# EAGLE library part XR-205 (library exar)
Monolithic WAVEFORM GENERATOR
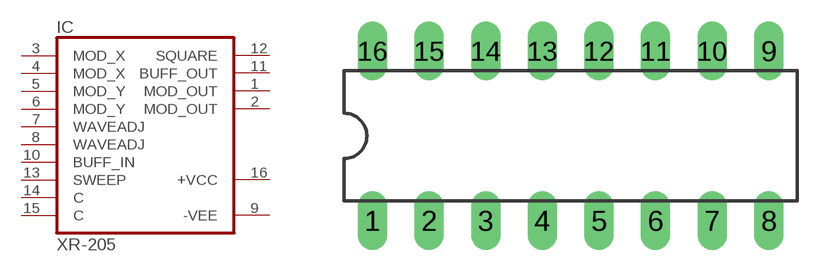
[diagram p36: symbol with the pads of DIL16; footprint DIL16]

Designator prefix IC

## XR-205 (OC_FARNELL: unknown; OC_NEWARK: unknown)  [DIL16]
1  MOD_OUT  out
2  MOD_OUT  out
3  MOD_X  in
4  MOD_X  in
5  MOD_Y  in
6  MOD_Y  in
7  WAVEADJ  in
8  WAVEADJ  in
9  -VEE  pwr
10  BUFF_IN  in
11  BUFF_OUT  out
12  SQUARE  out
13  SWEEP  in
14  C  in
15  C  in
16  +VCC  pwr

## Footprint DIL16 (pad centres in mm)
Dual In Line Package
drill 0.813 long: 1 -8.89,-3.81; 2 -6.35,-3.81; 3 -3.81,-3.81; 4 -1.27,-3.81; 5 1.27,-3.81; 6 3.81,-3.81; 7 6.35,-3.81; 8 8.89,-3.81; 9 8.89,3.81; 10 6.35,3.81; 11 3.81,3.81; 12 1.27,3.81; 13 -1.27,3.81; 14 -3.81,3.81; 15 -6.35,3.81; 16 -8.89,3.81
